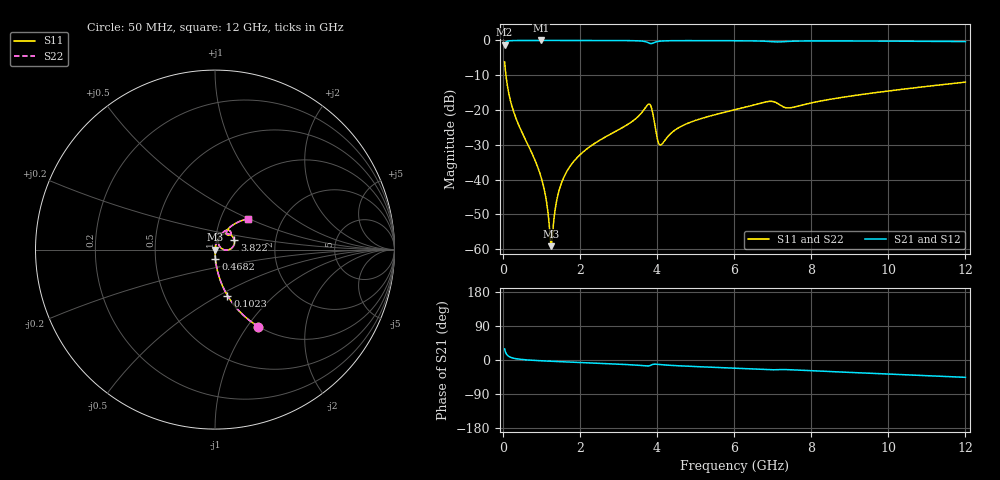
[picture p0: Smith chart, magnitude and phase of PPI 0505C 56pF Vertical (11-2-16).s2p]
# GHz S MA R 50
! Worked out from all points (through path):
!   1601 points, 50 MHz to 12 GHz, reference 50 ohm
!   highest |S21| = -0.01 dB at 991.1 MHz (marker M1); lowest = -1.2 dB at 50 MHz (marker M2)
!   group delay of S21, straight-line fit = 11 ps
!   lowest |S11| = -59.1 dB at 1.26 GHz (marker M3), VSWR 1.00, Z = 50.1 - j0.00641 ohm
!   |S11| at or under -10 dB: 84.7 MHz to end of sweep
!   |S22| runs from -59.1 to -6.2 dB; largest |S21 - S12| = 0
!   S11 on the Smith chart (normalised r, x): 50 MHz: 1.00, -1.13; 102.3 MHz: 1.00, -0.55; 468.2 MHz: 1.00, -0.10; 3.822 GHz: 1.23, +0.13; 12 GHz: 1.34, +0.49
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0.05  0.4925 -60.6  0.87 29.4  0.87 29.4  0.4925 -60.6
0.1022813  0.2654 -74.8  0.9638 15.1  0.9638 15.1  0.2654 -74.8
0.2367188  0.1148 -83.8  0.9928 6.0  0.9928 6.0  0.1148 -83.8
0.46825  0.05219 -87.5  0.9979 1.7  0.9979 1.7  0.05219 -87.5
0.9910625  0.01105 -86.9  0.9989 -2.0  0.9989 -2.0  0.01105 -86.9
1.110562  0.005854 -82.4  0.9989 -2.6  0.9989 -2.6  0.005854 -82.4
1.222594  0.001753 -54.8  0.9988 -3.2  0.9988 -3.2  0.001753 -54.8
1.259937  0.001105 -3.3  0.9988 -3.4  0.9988 -3.4  0.001105 -3.3
1.297281  0.001745 46.5  0.9988 -3.5  0.9988 -3.5  0.001745 46.5
1.409312  0.005287 73.2  0.9987 -4.1  0.9987 -4.1  0.005287 73.2
1.528812  0.009057 77.7  0.9986 -4.6  0.9986 -4.6  0.009057 77.7
2.044156  0.02381 79.7  0.9981 -6.8  0.9981 -6.8  0.02381 79.7
3.821719  0.1198 25.8  0.9055 -14.6  0.9055 -14.6  0.1198 25.8
4.038312  0.0341 16.0  0.9694 -11.6  0.9694 -11.6  0.0341 16.0
4.120469  0.03195 41.6  0.9807 -12.4  0.9807 -12.4  0.03195 41.6
4.807594  0.06467 69.6  0.9931 -16.5  0.9931 -16.5  0.06467 69.6
6.025  0.101 65.6  0.9898 -21.7  0.9898 -21.7  0.101 65.6
6.906313  0.133 53.3  0.9658 -25.7  0.9658 -25.7  0.133 53.3
7.39925  0.1071 50.2  0.9676 -25.5  0.9676 -25.5  0.1071 50.2
8.019156  0.1271 57.8  0.9829 -28.4  0.9829 -28.4  0.1271 57.8
10.01331  0.188 51.6  0.977 -37.0  0.977 -37.0  0.188 51.6
12  0.2516 43.2  0.9625 -45.7  0.9625 -45.7  0.2516 43.2
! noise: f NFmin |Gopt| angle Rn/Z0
0.05  0.000388  0.8643  0.4798  0.0006137
1.372  0.004018  0.6762  3.643  0.002392
2.701  0.007374  0.657  6.979  0.004087
4.031  0.03608  0.8814  10.7  0.06535
5.36  0.01448  0.6555  13.78  0.007902
6.682  0.02933  0.7735  17.4  0.02584
8.012  0.02637  0.7099  20.64  0.01734
9.341  0.02163  0.613  23.27  0.009979
10.67  0.02249  0.5849  26.03  0.009421
12  0.02434  0.5744  28.79  0.00977
